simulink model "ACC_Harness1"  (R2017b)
settings: Solver=FixedStepDiscrete  StartTime=0.0  StopTime=9  FixedStep=0.01  RelTol=1e-3  EnableMultiTasking=on
undefined symbols (not defined in the file): sigbuilder_block

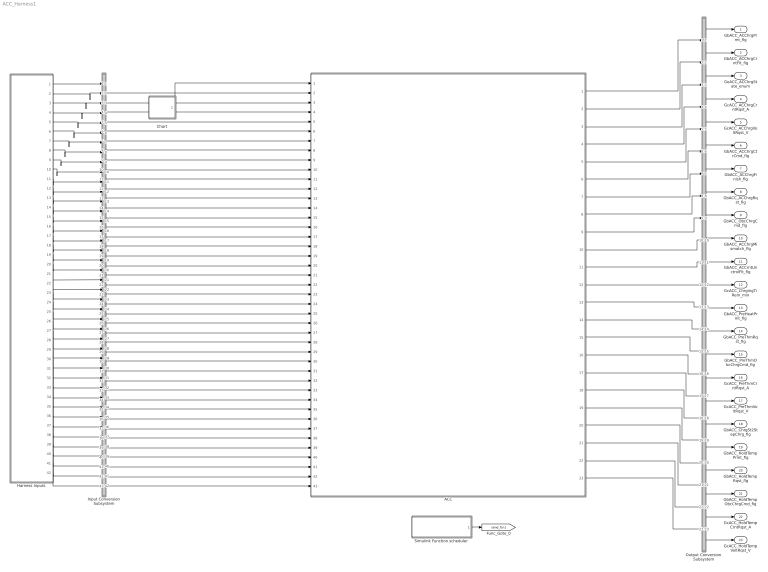
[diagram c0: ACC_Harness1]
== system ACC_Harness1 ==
  ACC : ModelReference  ModelNameDialog=ACC  SimulationMode=Normal  ModelReferenceVersion='M106C108'
  Chart : Stateflow chart  TreatAsAtomicUnit=on
  Harness Inputs : Subsystem  Tag=STV Subsys  LoadFcn=sigbuilder_block('load');  StartFcn=sigbuilder_block('start');  StopFcn=sigbuilder_block('stop');  ClipboardFcn=sigbuilder_block('clipboard');  mask(Sigbuilder block){tuvar=[0:10]}
      mask init:
      | if ~strcmp(get_param(bdroot(gcb),'SimulationStatus'),'stopped'),tuvar = sigbuilder_block('maskInit'); end
  Input Conversion Subsystem : Subsystem  Tag=__SLT_ICS__  Description=Signal spec. and routing
  Output Conversion Subsystem : Subsystem  Tag=__SLT_OCS__  Description=Signal spec. and routing
  Simulink Function scheduler : Test Sequence  Tag=__SLT_FCN_CALL__  TreatAsAtomicUnit=on
  GbACC_ACChrgPrmt_flg : Outport  OutDataTypeStr=boolean  PortDimensions=[1]
  GbACC_ACChrgCrntFlt_flg : Outport  Port=2  OutDataTypeStr=boolean  PortDimensions=[1]
  GeACC_ACChrgState_enum : Outport  Port=3  OutDataTypeStr=uint8  PortDimensions=[1]
  GcACC_ACChrgCrntRqst_A : Outport  Port=4  OutDataTypeStr=single  PortDimensions=[1]
  GcACC_ACChrgVoltRqst_V : Outport  Port=5  OutDataTypeStr=single  PortDimensions=[1]
  GbACC_ACChrgCtrCmd_flg : Outport  Port=6  OutDataTypeStr=boolean  PortDimensions=[1]
  GbACC_ACChrgFinish_flg : Outport  Port=7  OutDataTypeStr=boolean  PortDimensions=[1]
  GbACC_ACChrgRqst_flg : Outport  Port=8  OutDataTypeStr=boolean  PortDimensions=[1]
  GbACC_ObcChrgCmd_flg : Outport  Port=9  OutDataTypeStr=boolean  PortDimensions=[1]
  GbACC_ACChrgMismatch_flg : Outport  Port=10  OutDataTypeStr=boolean  PortDimensions=[1]
  GbACC_ACCrntUnctrolFlt_flg : Outport  Port=11  OutDataTypeStr=boolean  PortDimensions=[1]
  GcACC_ChrgingTiRem_min : Outport  Port=12  OutDataTypeStr=uint16  PortDimensions=[1]
  GbACC_PreHeatPrmt_flg : Outport  Port=13  OutDataTypeStr=boolean  PortDimensions=[1]
  GbACC_PreThmRqst_flg : Outport  Port=14  OutDataTypeStr=boolean  PortDimensions=[1]
  GbACC_PreThmObcChrgCmd_flg : Outport  Port=15  OutDataTypeStr=boolean  PortDimensions=[1]
  GcACC_PreThmCrntRqst_A : Outport  Port=16  OutDataTypeStr=single  PortDimensions=[1]
  GcACC_PreThmVoltRqst_V : Outport  Port=17  OutDataTypeStr=single  PortDimensions=[1]
  GbACC_ChrgSt2StepChrg_flg : Outport  Port=18  OutDataTypeStr=boolean  PortDimensions=[1]
  GbACC_HoldTempPrmt_flg : Outport  Port=19  OutDataTypeStr=boolean  PortDimensions=[1]
  GbACC_HoldTempRqst_flg : Outport  Port=20  OutDataTypeStr=boolean  PortDimensions=[1]
  GbACC_HoldTempObcChrgCmd_flg : Outport  Port=21  OutDataTypeStr=boolean  PortDimensions=[1]
  GcACC_HoldTempCrntRqst_A : Outport  Port=22  OutDataTypeStr=single  PortDimensions=[1]
  GcACC_HoldTempVoltRqst_V : Outport  Port=23  OutDataTypeStr=single  PortDimensions=[1]
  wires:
  Harness Inputs/1(GeBTM_HeatReq_enum) -> Input Conversion Subsystem/1(Inport_1)
  Harness Inputs/2(GeMSM_BMUState_enum) -> Input Conversion Subsystem/2(Inport_2)
  Harness Inputs/3(GeCTC_CtrCtlState_enum) -> Input Conversion Subsystem/3(Inport_3)
  Harness Inputs/4(GeCTC_CtrCtlConnMode_enum) -> Input Conversion Subsystem/4(Inport_4)
  Harness Inputs/5(GcODP_MaxCurrObcChrg_A) -> Input Conversion Subsystem/5(Inport_5)
  Harness Inputs/6(GcODP_MaxVoltObcChrg_V) -> Input Conversion Subsystem/6(Inport_6)
  Harness Inputs/7(GcODP_CurrObcChrg_A) -> Input Conversion Subsystem/7(Inport_7)
  Harness Inputs/8(GbODP_ACChrgAllow_flg) -> Input Conversion Subsystem/8(Inport_8)
  Harness Inputs/9(GcSOP_MaxChrgCurr_A) -> Input Conversion Subsystem/9(Inport_9)
  Harness Inputs/10(GcCDP_MaxCellVolt_mV) -> Input Conversion Subsystem/10(Inport_10)
  Harness Inputs/11(GcCDP_MinCellTemp_C) -> Input Conversion Subsystem/11(Inport_11)
  Harness Inputs/12(GcVDP_ChrgLdReq_numb) -> Input Conversion Subsystem/12(Inport_12)
  Harness Inputs/13(GcHDP_PackVolt_V) -> Input Conversion Subsystem/13(Inport_13)
  Harness Inputs/14(GcSOC_DispSOC_pct) -> Input Conversion Subsystem/14(Inport_14)
  Harness Inputs/15(GbWSM_ACWkUpPrs_flg) -> Input Conversion Subsystem/15(Inport_15)
  Harness Inputs/16(GeVDP_ChrgRqst_enum) -> Input Conversion Subsystem/16(Inport_16)
  Harness Inputs/17(GeODP_ObcElecLck_enum) -> Input Conversion Subsystem/17(Inport_17)
  Harness Inputs/18(GbADP_ChrgStopActive_flg) -> Input Conversion Subsystem/18(Inport_18)
  Harness Inputs/19(GcODP_ObcFaultLvl_numb) -> Input Conversion Subsystem/19(Inport_19)
  Harness Inputs/20(GeVDP_VcuFalutLvl_enum) -> Input Conversion Subsystem/20(Inport_20)
  Harness Inputs/21(GcCDP_MaxCellTemp_C) -> Input Conversion Subsystem/21(Inport_21)
  Harness Inputs/22(GeODP_ObcChrgSt_enum) -> Input Conversion Subsystem/22(Inport_22)
  Harness Inputs/23(GeVDP_PreThmVcuPmt_enum) -> Input Conversion Subsystem/23(Inport_23)
  Harness Inputs/24(GeVDP_PreThmEna_enum) -> Input Conversion Subsystem/24(Inport_24)
  Harness Inputs/25(GcHDP_PackCrnt_A) -> Input Conversion Subsystem/25(Inport_25)
  Harness Inputs/26(GcSOC_PackSOC_pct) -> Input Conversion Subsystem/26(Inport_26)
  Harness Inputs/27(GeODP_ObcCcSt_enum) -> Input Conversion Subsystem/27(Inport_27)
  Harness Inputs/28(GcODP_ObcCpDuty_numb) -> Input Conversion Subsystem/28(Inport_28)
  Harness Inputs/29(GcODP_MaxPwrObcChrg_W) -> Input Conversion Subsystem/29(Inport_29)
  Harness Inputs/30(GbFTC_OpenContactor_flg) -> Input Conversion Subsystem/30(Inport_30)
  Harness Inputs/31(GbFTC_PowerDown_flg) -> Input Conversion Subsystem/31(Inport_31)
  Harness Inputs/32(GbVDP_VcuChrgDisable_flg) -> Input Conversion Subsystem/32(Inport_32)
  Harness Inputs/33(GeODP_ObcCpSt_enum) -> Input Conversion Subsystem/33(Inport_33)
  Harness Inputs/34(GeUDS_AreaSel_enum) -> Input Conversion Subsystem/34(Inport_34)
  Harness Inputs/35(GcUDS_FullChrgCutoffVolt_mV) -> Input Conversion Subsystem/35(Inport_35)
  Harness Inputs/36(GcUDS_BatEnergy_kWh) -> Input Conversion Subsystem/36(Inport_36)
  Harness Inputs/37(GeUDS_CapSel_enum) -> Input Conversion Subsystem/37(Inport_37)
  Harness Inputs/38(GeADP_RmPreThemalReq_enum) -> Input Conversion Subsystem/38(Inport_38)
  Harness Inputs/39(GcADP_RmPreThemalTime_min) -> Input Conversion Subsystem/39(Inport_39)
  Harness Inputs/40(GbWSM_Kl15WkUpPrs_flg) -> Input Conversion Subsystem/40(Inport_40)
  Harness Inputs/41(GbADP_StopChgReq_flg) -> Input Conversion Subsystem/41(Inport_41)
  Harness Inputs/42(GbFTC_InhACChrg_flg) -> Input Conversion Subsystem/42(Inport_42)
  Output Conversion Subsystem/1(Outport_1) -> GbACC_ACChrgPrmt_flg/1
  Output Conversion Subsystem/2(Outport_2) -> GbACC_ACChrgCrntFlt_flg/1
  Output Conversion Subsystem/3(Outport_3) -> GeACC_ACChrgState_enum/1
  Output Conversion Subsystem/4(Outport_4) -> GcACC_ACChrgCrntRqst_A/1
  Output Conversion Subsystem/5(Outport_5) -> GcACC_ACChrgVoltRqst_V/1
  Output Conversion Subsystem/6(Outport_6) -> GbACC_ACChrgCtrCmd_flg/1
  Output Conversion Subsystem/7(Outport_7) -> GbACC_ACChrgFinish_flg/1
  Output Conversion Subsystem/8(Outport_8) -> GbACC_ACChrgRqst_flg/1
  Output Conversion Subsystem/9(Outport_9) -> GbACC_ObcChrgCmd_flg/1
  Output Conversion Subsystem/10(Outport_10) -> GbACC_ACChrgMismatch_flg/1
  Output Conversion Subsystem/11(Outport_11) -> GbACC_ACCrntUnctrolFlt_flg/1
  Output Conversion Subsystem/12(Outport_12) -> GcACC_ChrgingTiRem_min/1
  Output Conversion Subsystem/13(Outport_13) -> GbACC_PreHeatPrmt_flg/1
  Output Conversion Subsystem/14(Outport_14) -> GbACC_PreThmRqst_flg/1
  Output Conversion Subsystem/15(Outport_15) -> GbACC_PreThmObcChrgCmd_flg/1
  Output Conversion Subsystem/16(Outport_16) -> GcACC_PreThmCrntRqst_A/1
  Output Conversion Subsystem/17(Outport_17) -> GcACC_PreThmVoltRqst_V/1
  Output Conversion Subsystem/18(Outport_18) -> GbACC_ChrgSt2StepChrg_flg/1
  Output Conversion Subsystem/19(Outport_19) -> GbACC_HoldTempPrmt_flg/1
  Output Conversion Subsystem/20(Outport_20) -> GbACC_HoldTempRqst_flg/1
  Output Conversion Subsystem/21(Outport_21) -> GbACC_HoldTempObcChrgCmd_flg/1
  Output Conversion Subsystem/22(Outport_22) -> GcACC_HoldTempCrntRqst_A/1
  Output Conversion Subsystem/23(Outport_23) -> GcACC_HoldTempVoltRqst_V/1
  Input Conversion Subsystem/2(Outport_2) -> ACC/2
  Input Conversion Subsystem/3(Outport_3) -> ACC/3
  Input Conversion Subsystem/4(Outport_4) -> ACC/4
  Input Conversion Subsystem/5(Outport_5) -> ACC/5
  Input Conversion Subsystem/6(Outport_6) -> ACC/6
  Input Conversion Subsystem/7(Outport_7) -> ACC/7
  Input Conversion Subsystem/8(Outport_8) -> ACC/8
  Input Conversion Subsystem/9(Outport_9) -> ACC/9
  Input Conversion Subsystem/10(Outport_10) -> ACC/10
  Input Conversion Subsystem/11(Outport_11) -> ACC/11
  Input Conversion Subsystem/12(Outport_12) -> ACC/12
  Input Conversion Subsystem/13(Outport_13) -> ACC/13
  Input Conversion Subsystem/14(Outport_14) -> ACC/14
  Input Conversion Subsystem/15(Outport_15) -> ACC/15
  Input Conversion Subsystem/16(Outport_16) -> ACC/16
  Input Conversion Subsystem/17(Outport_17) -> ACC/17
  Input Conversion Subsystem/18(Outport_18) -> ACC/18
  Input Conversion Subsystem/19(Outport_19) -> ACC/19
  Input Conversion Subsystem/20(Outport_20) -> ACC/20
  Input Conversion Subsystem/21(Outport_21) -> ACC/21
  Input Conversion Subsystem/22(Outport_22) -> ACC/22
  Input Conversion Subsystem/23(Outport_23) -> ACC/23
  Input Conversion Subsystem/24(Outport_24) -> ACC/24
  Input Conversion Subsystem/25(Outport_25) -> ACC/25
  Input Conversion Subsystem/26(Outport_26) -> ACC/26
  Input Conversion Subsystem/27(Outport_27) -> ACC/27
  Input Conversion Subsystem/28(Outport_28) -> ACC/28
  Input Conversion Subsystem/29(Outport_29) -> ACC/29
  Input Conversion Subsystem/30(Outport_30) -> ACC/30
  Input Conversion Subsystem/31(Outport_31) -> ACC/31
  Input Conversion Subsystem/32(Outport_32) -> ACC/32
  Input Conversion Subsystem/33(Outport_33) -> ACC/33
  Input Conversion Subsystem/34(Outport_34) -> ACC/34
  Input Conversion Subsystem/35(Outport_35) -> ACC/35
  Input Conversion Subsystem/36(Outport_36) -> ACC/36
  Input Conversion Subsystem/37(Outport_37) -> ACC/37
  Input Conversion Subsystem/38(Outport_38) -> ACC/38
  Input Conversion Subsystem/39(Outport_39) -> ACC/39
  Input Conversion Subsystem/40(Outport_40) -> ACC/40
  Input Conversion Subsystem/41(Outport_41) -> ACC/41
  Input Conversion Subsystem/42(Outport_42) -> ACC/42
  Input Conversion Subsystem/43(Outport_43) -> ACC/43
  ACC/1 -> Output Conversion Subsystem/1(Inport_1)
  ACC/2 -> Output Conversion Subsystem/2(Inport_2)
  ACC/3 -> Output Conversion Subsystem/3(Inport_3)
  ACC/4 -> Output Conversion Subsystem/4(Inport_4)
  ACC/5 -> Output Conversion Subsystem/5(Inport_5)
  ACC/6 -> Output Conversion Subsystem/6(Inport_6)
  ACC/7 -> Output Conversion Subsystem/7(Inport_7)
  ACC/8 -> Output Conversion Subsystem/8(Inport_8)
  ACC/9 -> Output Conversion Subsystem/9(Inport_9)
  ACC/10 -> Output Conversion Subsystem/10(Inport_10)
  ACC/11 -> Output Conversion Subsystem/11(Inport_11)
  ACC/12 -> Output Conversion Subsystem/12(Inport_12)
  ACC/13 -> Output Conversion Subsystem/13(Inport_13)
  ACC/14 -> Output Conversion Subsystem/14(Inport_14)
  ACC/15 -> Output Conversion Subsystem/15(Inport_15)
  ACC/16 -> Output Conversion Subsystem/16(Inport_16)
  ACC/17 -> Output Conversion Subsystem/17(Inport_17)
  ACC/18 -> Output Conversion Subsystem/18(Inport_18)
  ACC/19 -> Output Conversion Subsystem/19(Inport_19)
  ACC/20 -> Output Conversion Subsystem/20(Inport_20)
  ACC/21 -> Output Conversion Subsystem/21(Inport_21)
  ACC/22 -> Output Conversion Subsystem/22(Inport_22)
  ACC/23 -> Output Conversion Subsystem/23(Inport_23)
  Simulink Function scheduler/1(ACC_ACChrgCon_100ms()) -> [send_fcn1]
  Chart/1(Run100ms()) -> ACC/1

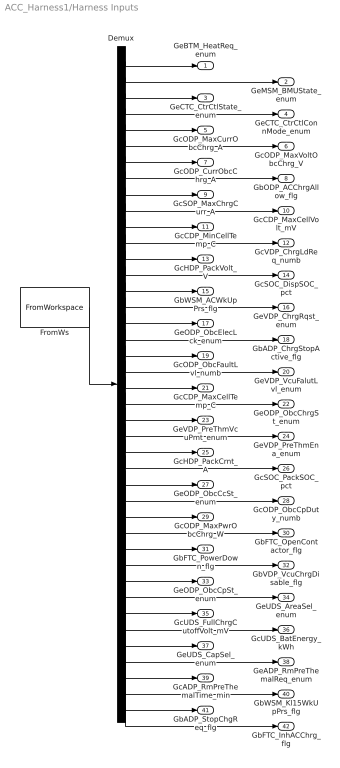
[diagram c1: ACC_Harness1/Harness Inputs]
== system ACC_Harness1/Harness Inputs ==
  Demux : Demux  Tag=STV Demux  Outputs=42
  FromWs : FromWorkspace  Tag=STV FromWs  VariableName=tuvar  SampleTime=0
  GeBTM_HeatReq_enum : Outport  Tag=STV Outport
  GeMSM_BMUState_enum : Outport  Tag=STV Outport  Port=2
  GeCTC_CtrCtlState_enum : Outport  Tag=STV Outport  Port=3
  GeCTC_CtrCtlConnMode_enum : Outport  Tag=STV Outport  Port=4
  GcODP_MaxCurrObcChrg_A : Outport  Tag=STV Outport  Port=5
  GcODP_MaxVoltObcChrg_V : Outport  Tag=STV Outport  Port=6
  GcODP_CurrObcChrg_A : Outport  Tag=STV Outport  Port=7
  GbODP_ACChrgAllow_flg : Outport  Tag=STV Outport  Port=8
  GcSOP_MaxChrgCurr_A : Outport  Tag=STV Outport  Port=9
  GcCDP_MaxCellVolt_mV : Outport  Tag=STV Outport  Port=10
  GcCDP_MinCellTemp_C : Outport  Tag=STV Outport  Port=11
  GcVDP_ChrgLdReq_numb : Outport  Tag=STV Outport  Port=12
  GcHDP_PackVolt_V : Outport  Tag=STV Outport  Port=13
  GcSOC_DispSOC_pct : Outport  Tag=STV Outport  Port=14
  GbWSM_ACWkUpPrs_flg : Outport  Tag=STV Outport  Port=15
  GeVDP_ChrgRqst_enum : Outport  Tag=STV Outport  Port=16
  GeODP_ObcElecLck_enum : Outport  Tag=STV Outport  Port=17
  GbADP_ChrgStopActive_flg : Outport  Tag=STV Outport  Port=18
  GcODP_ObcFaultLvl_numb : Outport  Tag=STV Outport  Port=19
  GeVDP_VcuFalutLvl_enum : Outport  Tag=STV Outport  Port=20
  GcCDP_MaxCellTemp_C : Outport  Tag=STV Outport  Port=21
  GeODP_ObcChrgSt_enum : Outport  Tag=STV Outport  Port=22
  GeVDP_PreThmVcuPmt_enum : Outport  Tag=STV Outport  Port=23
  GeVDP_PreThmEna_enum : Outport  Tag=STV Outport  Port=24
  GcHDP_PackCrnt_A : Outport  Tag=STV Outport  Port=25
  GcSOC_PackSOC_pct : Outport  Tag=STV Outport  Port=26
  GeODP_ObcCcSt_enum : Outport  Tag=STV Outport  Port=27
  GcODP_ObcCpDuty_numb : Outport  Tag=STV Outport  Port=28
  GcODP_MaxPwrObcChrg_W : Outport  Tag=STV Outport  Port=29
  GbFTC_OpenContactor_flg : Outport  Tag=STV Outport  Port=30
  GbFTC_PowerDown_flg : Outport  Tag=STV Outport  Port=31
  GbVDP_VcuChrgDisable_flg : Outport  Tag=STV Outport  Port=32
  GeODP_ObcCpSt_enum : Outport  Tag=STV Outport  Port=33
  GeUDS_AreaSel_enum : Outport  Tag=STV Outport  Port=34
  GcUDS_FullChrgCutoffVolt_mV : Outport  Tag=STV Outport  Port=35
  GcUDS_BatEnergy_kWh : Outport  Tag=STV Outport  Port=36
  GeUDS_CapSel_enum : Outport  Tag=STV Outport  Port=37
  GeADP_RmPreThemalReq_enum : Outport  Tag=STV Outport  Port=38
  GcADP_RmPreThemalTime_min : Outport  Tag=STV Outport  Port=39
  GbWSM_Kl15WkUpPrs_flg : Outport  Tag=STV Outport  Port=40
  GbADP_StopChgReq_flg : Outport  Tag=STV Outport  Port=41
  GbFTC_InhACChrg_flg : Outport  Tag=STV Outport  Port=42
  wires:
  FromWs/1 -> Demux/1
  Demux/1 -> GeBTM_HeatReq_enum/1
  Demux/2 -> GeMSM_BMUState_enum/1
  Demux/3 -> GeCTC_CtrCtlState_enum/1
  Demux/4 -> GeCTC_CtrCtlConnMode_enum/1
  Demux/5 -> GcODP_MaxCurrObcChrg_A/1
  Demux/6 -> GcODP_MaxVoltObcChrg_V/1
  Demux/7 -> GcODP_CurrObcChrg_A/1
  Demux/8 -> GbODP_ACChrgAllow_flg/1
  Demux/9 -> GcSOP_MaxChrgCurr_A/1
  Demux/10 -> GcCDP_MaxCellVolt_mV/1
  Demux/11 -> GcCDP_MinCellTemp_C/1
  Demux/12 -> GcVDP_ChrgLdReq_numb/1
  Demux/13 -> GcHDP_PackVolt_V/1
  Demux/14 -> GcSOC_DispSOC_pct/1
  Demux/15 -> GbWSM_ACWkUpPrs_flg/1
  Demux/16 -> GeVDP_ChrgRqst_enum/1
  Demux/17 -> GeODP_ObcElecLck_enum/1
  Demux/18 -> GbADP_ChrgStopActive_flg/1
  Demux/19 -> GcODP_ObcFaultLvl_numb/1
  Demux/20 -> GeVDP_VcuFalutLvl_enum/1
  Demux/21 -> GcCDP_MaxCellTemp_C/1
  Demux/22 -> GeODP_ObcChrgSt_enum/1
  Demux/23 -> GeVDP_PreThmVcuPmt_enum/1
  Demux/24 -> GeVDP_PreThmEna_enum/1
  Demux/25 -> GcHDP_PackCrnt_A/1
  Demux/26 -> GcSOC_PackSOC_pct/1
  Demux/27 -> GeODP_ObcCcSt_enum/1
  Demux/28 -> GcODP_ObcCpDuty_numb/1
  Demux/29 -> GcODP_MaxPwrObcChrg_W/1
  Demux/30 -> GbFTC_OpenContactor_flg/1
  Demux/31 -> GbFTC_PowerDown_flg/1
  Demux/32 -> GbVDP_VcuChrgDisable_flg/1
  Demux/33 -> GeODP_ObcCpSt_enum/1
  Demux/34 -> GeUDS_AreaSel_enum/1
  Demux/35 -> GcUDS_FullChrgCutoffVolt_mV/1
  Demux/36 -> GcUDS_BatEnergy_kWh/1
  Demux/37 -> GeUDS_CapSel_enum/1
  Demux/38 -> GeADP_RmPreThemalReq_enum/1
  Demux/39 -> GcADP_RmPreThemalTime_min/1
  Demux/40 -> GbWSM_Kl15WkUpPrs_flg/1
  Demux/41 -> GbADP_StopChgReq_flg/1
  Demux/42 -> GbFTC_InhACChrg_flg/1

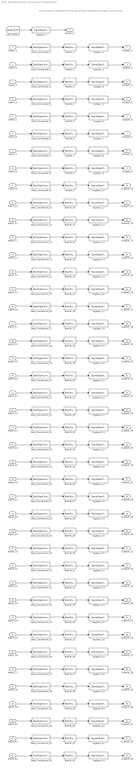
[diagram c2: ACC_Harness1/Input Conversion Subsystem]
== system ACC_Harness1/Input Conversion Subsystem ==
  note: This subsystem has been inserted by Simulink to adapt the output of the source blocks to the interface required by the harnessed component. Modifying the contents of this subsystem may result in compilation and simulation failure.
  Inport_1 : Inport
  Inport_2 : Inport  Port=2
  Inport_3 : Inport  Port=3
  Inport_4 : Inport  Port=4
  Inport_5 : Inport  Port=5
  Inport_6 : Inport  Port=6
  Inport_7 : Inport  Port=7
  Inport_8 : Inport  Port=8
  Inport_9 : Inport  Port=9
  Inport_10 : Inport  Port=10
  Inport_11 : Inport  Port=11
  Inport_12 : Inport  Port=12
  Inport_13 : Inport  Port=13
  Inport_14 : Inport  Port=14
  Inport_15 : Inport  Port=15
  Inport_16 : Inport  Port=16
  Inport_17 : Inport  Port=17
  Inport_18 : Inport  Port=18
  Inport_19 : Inport  Port=19
  Inport_20 : Inport  Port=20
  Inport_21 : Inport  Port=21
  Inport_22 : Inport  Port=22
  Inport_23 : Inport  Port=23
  Inport_24 : Inport  Port=24
  Inport_25 : Inport  Port=25
  Inport_26 : Inport  Port=26
  Inport_27 : Inport  Port=27
  Inport_28 : Inport  Port=28
  Inport_29 : Inport  Port=29
  Inport_30 : Inport  Port=30
  Inport_31 : Inport  Port=31
  Inport_32 : Inport  Port=32
  Inport_33 : Inport  Port=33
  Inport_34 : Inport  Port=34
  Inport_35 : Inport  Port=35
  Inport_36 : Inport  Port=36
  Inport_37 : Inport  Port=37
  Inport_38 : Inport  Port=38
  Inport_39 : Inport  Port=39
  Inport_40 : Inport  Port=40
  Inport_41 : Inport  Port=41
  Inport_42 : Inport  Port=42
  Data_Conversion_{1..4,16..17,19..20,22..24,27..28,33..34,37..38} (17 alike) : DataTypeConversion  OutDataTypeStr=uint8
  Data_Conversion_{10,29,35..36} (4 alike) : DataTypeConversion  OutDataTypeStr=uint16
  Data_Conversion_{5..7,9,11..14,21,25..26,39} (12 alike) : DataTypeConversion  OutDataTypeStr=single
  Data_Conversion_{8,15,18,30..32,40..42} (9 alike) : DataTypeConversion  OutDataTypeStr=boolean
  RateTs_{1..42} (42 alike) : RateTransition
  SigSpec_1 : SignalSpecification
  SigSpec_{6,8,10,26} (4 alike) : SignalSpecification  OutDataTypeStr=single  Unit=A  Dimensions=[1]
  SigSpec_11 : SignalSpecification  OutDataTypeStr=uint16  Unit=mV  Dimensions=[1]
  SigSpec_12 : SignalSpecification  OutDataTypeStr=single  Unit=C  Dimensions=[1]
  SigSpec_13 : SignalSpecification  OutDataTypeStr=single  Unit=kW  Dimensions=[1]
  SigSpec_14 : SignalSpecification  OutDataTypeStr=single  Unit=V  Dimensions=[1]
  SigSpec_15 : SignalSpecification  OutDataTypeStr=single  Unit=pct  Dimensions=[1]
  SigSpec_{16,19,33,41} (4 alike) : SignalSpecification  OutDataTypeStr=boolean  Unit=flg  Dimensions=[1]
  SigSpec_{2..5,17,21,24..25,35,38..39} (11 alike) : SignalSpecification  OutDataTypeStr=uint8  Unit=enum  Dimensions=[1]
  SigSpec_{18,20,23,28,34} (5 alike) : SignalSpecification  OutDataTypeStr=uint8  Unit=numb  Dimensions=[1]
  SigSpec_22 : SignalSpecification  OutDataTypeStr=single  Unit=C  Dimensions=[1]
  SigSpec_27 : SignalSpecification  OutDataTypeStr=single  Unit=pct  Dimensions=[1]
  SigSpec_29 : SignalSpecification  OutDataTypeStr=uint8  Unit=%  Dimensions=[1]
  SigSpec_30 : SignalSpecification  OutDataTypeStr=uint16  Unit=W  Dimensions=[1]
  SigSpec_{9,31..32,42..43} (5 alike) : SignalSpecification  OutDataTypeStr=boolean  Unit=flag  Dimensions=[1]
  SigSpec_36 : SignalSpecification  OutDataTypeStr=uint16  Unit=mV  Dimensions=[1]
  SigSpec_37 : SignalSpecification  OutDataTypeStr=uint16  Unit=kWh  Dimensions=[1]
  SigSpec_40 : SignalSpecification  OutDataTypeStr=single  Unit=min  Dimensions=[1]
  SigSpec_7 : SignalSpecification  OutDataTypeStr=single  Unit=V  Dimensions=[1]
  Outport_1 : Outport
  Outport_2 : Outport  Port=2
  Outport_3 : Outport  Port=3
  Outport_4 : Outport  Port=4
  Outport_5 : Outport  Port=5
  Outport_6 : Outport  Port=6
  Outport_7 : Outport  Port=7
  Outport_8 : Outport  Port=8
  Outport_9 : Outport  Port=9
  Outport_10 : Outport  Port=10
  Outport_11 : Outport  Port=11
  Outport_12 : Outport  Port=12
  Outport_13 : Outport  Port=13
  Outport_14 : Outport  Port=14
  Outport_15 : Outport  Port=15
  Outport_16 : Outport  Port=16
  Outport_17 : Outport  Port=17
  Outport_18 : Outport  Port=18
  Outport_19 : Outport  Port=19
  Outport_20 : Outport  Port=20
  Outport_21 : Outport  Port=21
  Outport_22 : Outport  Port=22
  Outport_23 : Outport  Port=23
  Outport_24 : Outport  Port=24
  Outport_25 : Outport  Port=25
  Outport_26 : Outport  Port=26
  Outport_27 : Outport  Port=27
  Outport_28 : Outport  Port=28
  Outport_29 : Outport  Port=29
  Outport_30 : Outport  Port=30
  Outport_31 : Outport  Port=31
  Outport_32 : Outport  Port=32
  Outport_33 : Outport  Port=33
  Outport_34 : Outport  Port=34
  Outport_35 : Outport  Port=35
  Outport_36 : Outport  Port=36
  Outport_37 : Outport  Port=37
  Outport_38 : Outport  Port=38
  Outport_39 : Outport  Port=39
  Outport_40 : Outport  Port=40
  Outport_41 : Outport  Port=41
  Outport_42 : Outport  Port=42
  Outport_43 : Outport  Port=43
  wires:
  SigSpec_1/1 -> Outport_1/1
  [send_fcn1] -> SigSpec_1/1
  SigSpec_2/1 -> Outport_2/1
  RateTs_1/1 -> SigSpec_2/1
  Data_Conversion_1/1 -> RateTs_1/1
  Inport_1/1 -> Data_Conversion_1/1
  SigSpec_3/1 -> Outport_3/1
  RateTs_2/1 -> SigSpec_3/1
  Data_Conversion_2/1 -> RateTs_2/1
  Inport_2/1 -> Data_Conversion_2/1
  SigSpec_4/1 -> Outport_4/1
  RateTs_3/1 -> SigSpec_4/1
  Data_Conversion_3/1 -> RateTs_3/1
  Inport_3/1 -> Data_Conversion_3/1
  SigSpec_5/1 -> Outport_5/1
  RateTs_4/1 -> SigSpec_5/1
  Data_Conversion_4/1 -> RateTs_4/1
  Inport_4/1 -> Data_Conversion_4/1
  SigSpec_6/1 -> Outport_6/1
  RateTs_5/1 -> SigSpec_6/1
  Data_Conversion_5/1 -> RateTs_5/1
  Inport_5/1 -> Data_Conversion_5/1
  SigSpec_7/1 -> Outport_7/1
  RateTs_6/1 -> SigSpec_7/1
  Data_Conversion_6/1 -> RateTs_6/1
  Inport_6/1 -> Data_Conversion_6/1
  SigSpec_8/1 -> Outport_8/1
  RateTs_7/1 -> SigSpec_8/1
  Data_Conversion_7/1 -> RateTs_7/1
  Inport_7/1 -> Data_Conversion_7/1
  SigSpec_9/1 -> Outport_9/1
  RateTs_8/1 -> SigSpec_9/1
  Data_Conversion_8/1 -> RateTs_8/1
  Inport_8/1 -> Data_Conversion_8/1
  SigSpec_10/1 -> Outport_10/1
  RateTs_9/1 -> SigSpec_10/1
  Data_Conversion_9/1 -> RateTs_9/1
  Inport_9/1 -> Data_Conversion_9/1
  SigSpec_11/1 -> Outport_11/1
  RateTs_10/1 -> SigSpec_11/1
  Data_Conversion_10/1 -> RateTs_10/1
  Inport_10/1 -> Data_Conversion_10/1
  SigSpec_12/1 -> Outport_12/1
  RateTs_11/1 -> SigSpec_12/1
  Data_Conversion_11/1 -> RateTs_11/1
  Inport_11/1 -> Data_Conversion_11/1
  SigSpec_13/1 -> Outport_13/1
  RateTs_12/1 -> SigSpec_13/1
  Data_Conversion_12/1 -> RateTs_12/1
  Inport_12/1 -> Data_Conversion_12/1
  SigSpec_14/1 -> Outport_14/1
  RateTs_13/1 -> SigSpec_14/1
  Data_Conversion_13/1 -> RateTs_13/1
  Inport_13/1 -> Data_Conversion_13/1
  SigSpec_15/1 -> Outport_15/1
  RateTs_14/1 -> SigSpec_15/1
  Data_Conversion_14/1 -> RateTs_14/1
  Inport_14/1 -> Data_Conversion_14/1
  SigSpec_16/1 -> Outport_16/1
  RateTs_15/1 -> SigSpec_16/1
  Data_Conversion_15/1 -> RateTs_15/1
  Inport_15/1 -> Data_Conversion_15/1
  SigSpec_17/1 -> Outport_17/1
  RateTs_16/1 -> SigSpec_17/1
  Data_Conversion_16/1 -> RateTs_16/1
  Inport_16/1 -> Data_Conversion_16/1
  SigSpec_18/1 -> Outport_18/1
  RateTs_17/1 -> SigSpec_18/1
  Data_Conversion_17/1 -> RateTs_17/1
  Inport_17/1 -> Data_Conversion_17/1
  SigSpec_19/1 -> Outport_19/1
  RateTs_18/1 -> SigSpec_19/1
  Data_Conversion_18/1 -> RateTs_18/1
  Inport_18/1 -> Data_Conversion_18/1
  SigSpec_20/1 -> Outport_20/1
  RateTs_19/1 -> SigSpec_20/1
  Data_Conversion_19/1 -> RateTs_19/1
  Inport_19/1 -> Data_Conversion_19/1
  SigSpec_21/1 -> Outport_21/1
  RateTs_20/1 -> SigSpec_21/1
  Data_Conversion_20/1 -> RateTs_20/1
  Inport_20/1 -> Data_Conversion_20/1
  SigSpec_22/1 -> Outport_22/1
  RateTs_21/1 -> SigSpec_22/1
  Data_Conversion_21/1 -> RateTs_21/1
  Inport_21/1 -> Data_Conversion_21/1
  SigSpec_23/1 -> Outport_23/1
  RateTs_22/1 -> SigSpec_23/1
  Data_Conversion_22/1 -> RateTs_22/1
  Inport_22/1 -> Data_Conversion_22/1
  SigSpec_24/1 -> Outport_24/1
  RateTs_23/1 -> SigSpec_24/1
  Data_Conversion_23/1 -> RateTs_23/1
  Inport_23/1 -> Data_Conversion_23/1
  SigSpec_25/1 -> Outport_25/1
  RateTs_24/1 -> SigSpec_25/1
  Data_Conversion_24/1 -> RateTs_24/1
  Inport_24/1 -> Data_Conversion_24/1
  SigSpec_26/1 -> Outport_26/1
  RateTs_25/1 -> SigSpec_26/1
  Data_Conversion_25/1 -> RateTs_25/1
  Inport_25/1 -> Data_Conversion_25/1
  SigSpec_27/1 -> Outport_27/1
  RateTs_26/1 -> SigSpec_27/1
  Data_Conversion_26/1 -> RateTs_26/1
  Inport_26/1 -> Data_Conversion_26/1
  SigSpec_28/1 -> Outport_28/1
  RateTs_27/1 -> SigSpec_28/1
  Data_Conversion_27/1 -> RateTs_27/1
  Inport_27/1 -> Data_Conversion_27/1
  SigSpec_29/1 -> Outport_29/1
  RateTs_28/1 -> SigSpec_29/1
  Data_Conversion_28/1 -> RateTs_28/1
  Inport_28/1 -> Data_Conversion_28/1
  SigSpec_30/1 -> Outport_30/1
  RateTs_29/1 -> SigSpec_30/1
  Data_Conversion_29/1 -> RateTs_29/1
  Inport_29/1 -> Data_Conversion_29/1
  SigSpec_31/1 -> Outport_31/1
  RateTs_30/1 -> SigSpec_31/1
  Data_Conversion_30/1 -> RateTs_30/1
  Inport_30/1 -> Data_Conversion_30/1
  SigSpec_32/1 -> Outport_32/1
  RateTs_31/1 -> SigSpec_32/1
  Data_Conversion_31/1 -> RateTs_31/1
  Inport_31/1 -> Data_Conversion_31/1
  SigSpec_33/1 -> Outport_33/1
  RateTs_32/1 -> SigSpec_33/1
  Data_Conversion_32/1 -> RateTs_32/1
  Inport_32/1 -> Data_Conversion_32/1
  SigSpec_34/1 -> Outport_34/1
  RateTs_33/1 -> SigSpec_34/1
  Data_Conversion_33/1 -> RateTs_33/1
  Inport_33/1 -> Data_Conversion_33/1
  SigSpec_35/1 -> Outport_35/1
  RateTs_34/1 -> SigSpec_35/1
  Data_Conversion_34/1 -> RateTs_34/1
  Inport_34/1 -> Data_Conversion_34/1
  SigSpec_36/1 -> Outport_36/1
  RateTs_35/1 -> SigSpec_36/1
  Data_Conversion_35/1 -> RateTs_35/1
  Inport_35/1 -> Data_Conversion_35/1
  SigSpec_37/1 -> Outport_37/1
  RateTs_36/1 -> SigSpec_37/1
  Data_Conversion_36/1 -> RateTs_36/1
  Inport_36/1 -> Data_Conversion_36/1
  SigSpec_38/1 -> Outport_38/1
  RateTs_37/1 -> SigSpec_38/1
  Data_Conversion_37/1 -> RateTs_37/1
  Inport_37/1 -> Data_Conversion_37/1
  SigSpec_39/1 -> Outport_39/1
  RateTs_38/1 -> SigSpec_39/1
  Data_Conversion_38/1 -> RateTs_38/1
  Inport_38/1 -> Data_Conversion_38/1
  SigSpec_40/1 -> Outport_40/1
  RateTs_39/1 -> SigSpec_40/1
  Data_Conversion_39/1 -> RateTs_39/1
  Inport_39/1 -> Data_Conversion_39/1
  SigSpec_41/1 -> Outport_41/1
  RateTs_40/1 -> SigSpec_41/1
  Data_Conversion_40/1 -> RateTs_40/1
  Inport_40/1 -> Data_Conversion_40/1
  SigSpec_42/1 -> Outport_42/1
  RateTs_41/1 -> SigSpec_42/1
  Data_Conversion_41/1 -> RateTs_41/1
  Inport_41/1 -> Data_Conversion_41/1
  SigSpec_43/1 -> Outport_43/1
  RateTs_42/1 -> SigSpec_43/1
  Data_Conversion_42/1 -> RateTs_42/1
  Inport_42/1 -> Data_Conversion_42/1

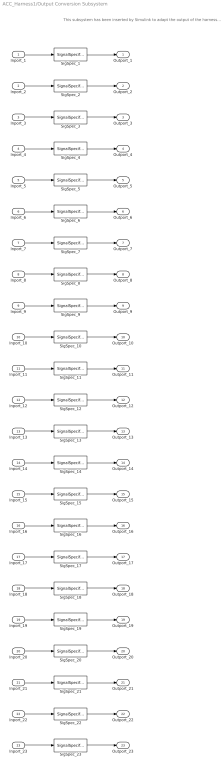
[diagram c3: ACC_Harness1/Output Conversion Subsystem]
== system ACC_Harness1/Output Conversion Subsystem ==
  note: This subsystem has been inserted by Simulink to adapt the output of the harnessed component to the interface required by the sink blocks. Modifying the contents of this subsystem may result in compilation and simulation failure.
  Inport_1 : Inport
  Inport_2 : Inport  Port=2
  Inport_3 : Inport  Port=3
  Inport_4 : Inport  Port=4
  Inport_5 : Inport  Port=5
  Inport_6 : Inport  Port=6
  Inport_7 : Inport  Port=7
  Inport_8 : Inport  Port=8
  Inport_9 : Inport  Port=9
  Inport_10 : Inport  Port=10
  Inport_11 : Inport  Port=11
  Inport_12 : Inport  Port=12
  Inport_13 : Inport  Port=13
  Inport_14 : Inport  Port=14
  Inport_15 : Inport  Port=15
  Inport_16 : Inport  Port=16
  Inport_17 : Inport  Port=17
  Inport_18 : Inport  Port=18
  Inport_19 : Inport  Port=19
  Inport_20 : Inport  Port=20
  Inport_21 : Inport  Port=21
  Inport_22 : Inport  Port=22
  Inport_23 : Inport  Port=23
  SigSpec_{1..2,6..11,13..15,18..21} (15 alike) : SignalSpecification  OutDataTypeStr=boolean  Unit=flag  Dimensions=[1]
  SigSpec_12 : SignalSpecification  OutDataTypeStr=uint16  Unit=min  Dimensions=[1]
  SigSpec_16 : SignalSpecification  OutDataTypeStr=single  Unit=A  Dimensions=[1]
  SigSpec_17 : SignalSpecification  OutDataTypeStr=single  Unit=V  Dimensions=[1]
  SigSpec_22 : SignalSpecification  OutDataTypeStr=single  Unit=A  Dimensions=[1]
  SigSpec_23 : SignalSpecification  OutDataTypeStr=single  Unit=V  Dimensions=[1]
  SigSpec_3 : SignalSpecification  OutDataTypeStr=uint8  Unit=enum  Dimensions=[1]
  SigSpec_4 : SignalSpecification  OutDataTypeStr=single  Unit=A  Dimensions=[1]
  SigSpec_5 : SignalSpecification  OutDataTypeStr=single  Unit=V  Dimensions=[1]
  Outport_1 : Outport
  Outport_2 : Outport  Port=2
  Outport_3 : Outport  Port=3
  Outport_4 : Outport  Port=4
  Outport_5 : Outport  Port=5
  Outport_6 : Outport  Port=6
  Outport_7 : Outport  Port=7
  Outport_8 : Outport  Port=8
  Outport_9 : Outport  Port=9
  Outport_10 : Outport  Port=10
  Outport_11 : Outport  Port=11
  Outport_12 : Outport  Port=12
  Outport_13 : Outport  Port=13
  Outport_14 : Outport  Port=14
  Outport_15 : Outport  Port=15
  Outport_16 : Outport  Port=16
  Outport_17 : Outport  Port=17
  Outport_18 : Outport  Port=18
  Outport_19 : Outport  Port=19
  Outport_20 : Outport  Port=20
  Outport_21 : Outport  Port=21
  Outport_22 : Outport  Port=22
  Outport_23 : Outport  Port=23
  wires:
  Inport_1/1 -> SigSpec_1/1
  SigSpec_1/1 -> Outport_1/1
  Inport_2/1 -> SigSpec_2/1
  SigSpec_2/1 -> Outport_2/1
  Inport_3/1 -> SigSpec_3/1
  SigSpec_3/1 -> Outport_3/1
  Inport_4/1 -> SigSpec_4/1
  SigSpec_4/1 -> Outport_4/1
  Inport_5/1 -> SigSpec_5/1
  SigSpec_5/1 -> Outport_5/1
  Inport_6/1 -> SigSpec_6/1
  SigSpec_6/1 -> Outport_6/1
  Inport_7/1 -> SigSpec_7/1
  SigSpec_7/1 -> Outport_7/1
  Inport_8/1 -> SigSpec_8/1
  SigSpec_8/1 -> Outport_8/1
  Inport_9/1 -> SigSpec_9/1
  SigSpec_9/1 -> Outport_9/1
  Inport_10/1 -> SigSpec_10/1
  SigSpec_10/1 -> Outport_10/1
  Inport_11/1 -> SigSpec_11/1
  SigSpec_11/1 -> Outport_11/1
  Inport_12/1 -> SigSpec_12/1
  SigSpec_12/1 -> Outport_12/1
  Inport_13/1 -> SigSpec_13/1
  SigSpec_13/1 -> Outport_13/1
  Inport_14/1 -> SigSpec_14/1
  SigSpec_14/1 -> Outport_14/1
  Inport_15/1 -> SigSpec_15/1
  SigSpec_15/1 -> Outport_15/1
  Inport_16/1 -> SigSpec_16/1
  SigSpec_16/1 -> Outport_16/1
  Inport_17/1 -> SigSpec_17/1
  SigSpec_17/1 -> Outport_17/1
  Inport_18/1 -> SigSpec_18/1
  SigSpec_18/1 -> Outport_18/1
  Inport_19/1 -> SigSpec_19/1
  SigSpec_19/1 -> Outport_19/1
  Inport_20/1 -> SigSpec_20/1
  SigSpec_20/1 -> Outport_20/1
  Inport_21/1 -> SigSpec_21/1
  SigSpec_21/1 -> Outport_21/1
  Inport_22/1 -> SigSpec_22/1
  SigSpec_22/1 -> Outport_22/1
  Inport_23/1 -> SigSpec_23/1
  SigSpec_23/1 -> Outport_23/1

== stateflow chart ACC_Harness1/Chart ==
  (default) -> (junction 1)
  (junction 1) -> (junction 3) : {Run100ms}
  events: output FUNCTION_CALL_EVENT

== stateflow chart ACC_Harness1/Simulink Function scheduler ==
  state Run
  state AsyncFunctionCalls
    % Call Asynchronous FunctionCall Subsystems.
    %
    %% Schedule function-call outputs.
    %% Modify this code to change function-call order.
    send(ACC_ACChrgCon_100ms)
  (default) -> Run
  events: output FUNCTION_CALL_EVENT
